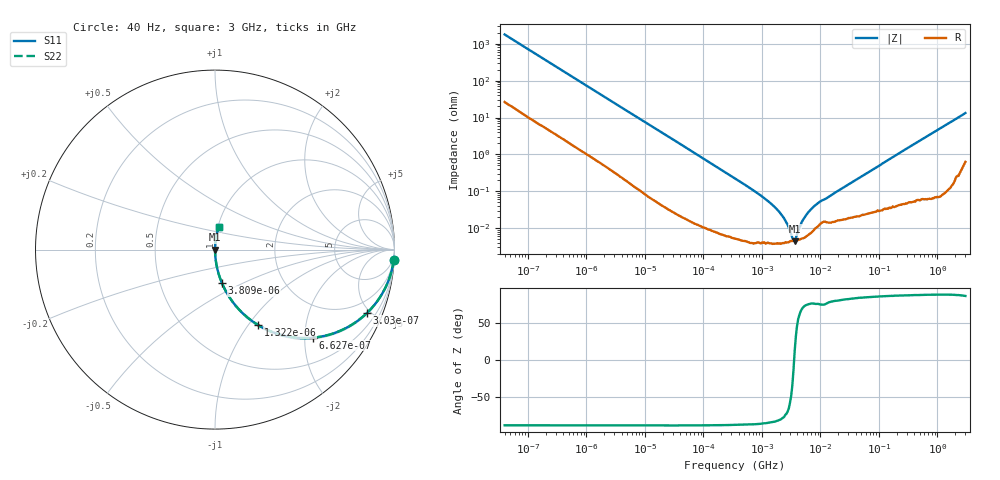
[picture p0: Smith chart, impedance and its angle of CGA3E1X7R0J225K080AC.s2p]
! S-parameter Generated by TDK Corporation
! Copyright(C) 2015 TDK Corporation.
! All Rights Reserved.
! TDK P/N: CGA3E1X7R0J225K080AC (Multilayer Ceramic Chip Capacitors)
! Property: C=2.2uF
! Size(LxWxT): 1.6x0.8x0.8mm, 0.063x0.031x0.031inches
! Model Type: s2p (Touchstone File Format Version 1.0)
! Frequency: DC=Yes Start=0.00004MHz Stop=3000MHz 396points Log-sweep
! Note: This model was converted from impedance.
! Model Generated on Jun. 23, 2015
! Hash(MD5):
! Port Assignments:
!  1 ---| |--- 2
! Applicable Conditions:
!  Temperature = 25 degC
!  DC Bias Voltage = 0 V
!  Small Signal Operation
! Terms and conditions regarding TDK Simulation Models
! (1)This simulation model is being provided solely for informational purposes. Please refer to the specifications of the products in terms of detailed characteristics of such products.
! (2)In no event shall TDK Corporation of any of its subsidiaries be liable for any loss or damage arising, directly or indirectly,
!  From any information contained in this simulation model, including, but not limited to loss or damages arising from any inaccuracies, omissions or errors in connection with such information.
! (3)Any and all copyrights on this simulation model are owned by TDK Corporation.
!  Duplication or redistribution of this simulation model without prior written permission from TDK Corporation is prohibited.
! (4)This simulation model is subject to any modification or change without any prior notice.
! (5)Neither TDK Corporation nor any of its subsidiaries shall make any warranty, express or implied,
!  Including but not limited to the correctness, implied warranties of merchantability and fitness for a particular purpose with respect to this simulation models.
! (6)The use of this simulation model shall be deemed to have consented to the terms and conditions hereof.
# MHz S MA R 50
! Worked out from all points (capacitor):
!   395 points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, 40 Hz to 3 GHz, reference 50 ohm
!   read as one part in series: C = 2.22 uF near 41.88 Hz
!   lowest |Z| = 4.43 mohm at 3.622 MHz (marker M1)
!   series resonance near 3.551 MHz, so ESL is about 900 pH
!   S11 on the Smith chart (normalised r, x): 40 Hz: 2, -36; 303 Hz: 1.07, -4.78; 662.7 Hz: 1.03, -2.20; 1.322 kHz: 1.02, -1.11; 3.809 kHz: 1.00, -0.39; 3 GHz: 1.01, +0.27
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4e-05  0.9976 -3.2  0.05571 86.0  0.05571 86.0  0.9976 -3.2
0.0001451139  0.9777 -11.3  0.1967 77.9  0.1967 77.9  0.9777 -11.3
0.0003030459  0.918 -22.6  0.3837 66.6  0.3837 66.6  0.918 -22.6
0.000662667  0.735 -41.9  0.6679 47.3  0.6679 47.3  0.735 -41.9
0.000834128  0.6544 -48.3  0.7472 40.9  0.7472 40.9  0.6544 -48.3
0.001321622  0.4826 -60.4  0.8692 28.9  0.8692 28.9  0.4826 -60.4
0.002192651  0.3176 -70.7  0.944 18.5  0.944 18.5  0.3176 -70.7
0.003809071  0.1912 -78.3  0.9792 11.0  0.9792 11.0  0.1912 -78.3
0.01739424  0.04374 -86.9  0.9986 2.5  0.9986 2.5  0.04374 -86.9
0.3464102  0.002235 -88.6  0.9999 0.1  0.9999 0.1  0.002235 -88.6
1.315913  0.0005157 -85.6  1 0.0  1 0.0  0.0005157 -85.6
2.183178  0.0002252 -80.1  1 0.0  1 0.0  0.0002252 -80.1
2.877491  0.0001028 -66.2  1 0.0  1 0.0  0.0001028 -66.2
3.622024  4.433e-05 11.5  1 -0.0  1 -0.0  4.433e-05 11.5
4.354128  0.0001006 61.1  1 -0.0  1 -0.0  0.0001006 61.1
4.773931  0.000144 68.9  0.9999 -0.0  0.9999 -0.0  0.000144 68.9
5.480732  0.0002078 74.3  0.9999 -0.0  0.9999 -0.0  0.0002078 74.3
7.22376  0.0003504 76.9  0.9999 -0.0  0.9999 -0.0  0.0003504 76.9
9.969551  0.0005302 75.7  0.9999 -0.0  0.9999 -0.0  0.0005302 75.7
150.6385  0.007398 86.8  0.9996 -0.4  0.9996 -0.4  0.007398 86.8
949.3681  0.04397 86.6  0.9983 -2.5  0.9983 -2.5  0.04397 86.6
3000  0.1307 79.8  0.9853 -7.5  0.9853 -7.5  0.1307 79.8
